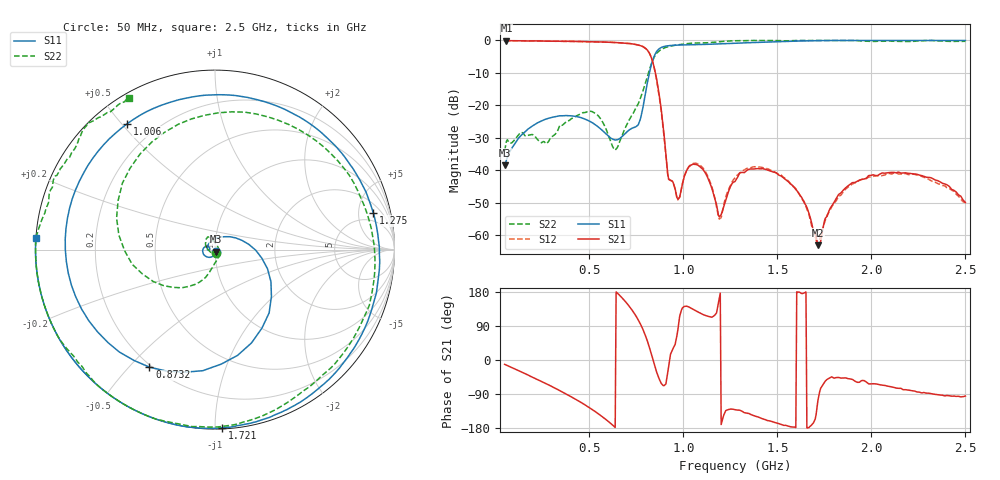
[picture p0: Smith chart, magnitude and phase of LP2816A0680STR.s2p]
!	AVX THIN FILM OPERATION
!	LP2816S High Performance Low Pass Filters
!	P/N LP2816S0680ANTR
! Created  22 November 2016
!Instrument: 	"HEWLETT PACKARD,8720ES,US39172150,7.62 "
# MHz S dB R 50
!  Frq	S11(dB)	S11(deg)	S21(dB)	S21(deg)	S12(dB)	S12(deg)	S22(dB)	S22(deg)
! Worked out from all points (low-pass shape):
!   501 points, 50 MHz to 2.5 GHz, reference 50 ohm
!   highest |S21| = -0.06 dB at 59.8 MHz (marker M1); lowest = -63.1 dB at 1.716 GHz (marker M2)
!   |S21| within 3 dB of the highest: start of sweep to 810.4 MHz
!   lowest |S11| = -38.5 dB at 50 MHz (marker M3), VSWR 1.02, Z = 50.5 - j1.1 ohm
!   |S11| at or under -10 dB: start of sweep to 819.8 MHz
!   |S22| runs from -34.0 to 0.0 dB; largest |S21 - S12| = 0.015
!   S11 on the Smith chart (normalised r, x): 50 MHz: 1.01, -0.02; 873.2 MHz: 0.19, -0.57; 1.006 GHz: 0.10, +0.52; 1.275 GHz: 3.24, +7.36; 1.721 GHz: 0.01, -1.04; 2.5 GHz: -0.00, +0.03
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50  -38.47 -65.8  -0.06 -11.4  -0.07 -11.4  -33.97 -65.4
59.8  -36.78 -73.9  -0.06 -13.5  -0.07 -13.7  -31.05 -76.1
221.5  -25.46 -125.7  -0.14 -50.7  -0.16 -50.6  -30.28 -90.4
461.6  -23.87 172.2  -0.34 -113.5  -0.35 -113.6  -22.38 130.3
642.9  -30.62 174.9  -0.65 179.7  -0.65 179.5  -33.45 8.4
760.5  -25.97 116.5  -1.40 105.9  -1.40 105.4  -19.52 -99.6
819.3  -10.13 -20.1  -3.85 34.1  -3.89 32.9  -9.13 -144.9
868.3  -2.75 -111.8  -15.38 -45.7  -15.77 -46.7  -3.39 128.1
873.2  -2.50 -119.2  -17.25 -51.6  -17.69 -52.4  -3.16 120.5
927.1  -1.58 -179.7  -42.87 -1.2  -42.91 1.8  -1.84 59.4
971.2  -1.42 146.5  -48.88 79.6  -49.08 81.5  -1.33 25.7
1005.5  -1.36 124.9  -41.87 141.4  -41.72 144.8  -1.09 4.6
1103.5  -1.24 75.8  -39.64 120.1  -39.19 121.9  -0.73 -39.8
1196.6  -1.05 39.1  -54.00 176.5  -54.77 178.2  -0.36 -72.3
1275  -0.86 13.0  -43.43 -131.2  -42.27 -132.4  -0.09 -92.0
1520  -0.33 -49.9  -41.73 -170.1  -41.44 -172.3  -0.06 -136.2
1686.6  -0.10 -81.9  -57.29 -169.0  -58.00 -174.1  0.00 -160.0
1716  -0.07 -86.9  -63.12 -106.2  -63.34 -116.6  0.00 -163.8
1720.9  -0.06 -87.7  -62.92 -94.3  -62.27 -106.4  0.00 -164.4
1833.6  0.00 -105.5  -47.10 -47.1  -47.79 -52.0  0.00 -177.3
2093.3  0.00 -140.3  -40.70 -69.5  -40.94 -70.8  -0.16 155.7
2500  0.00 176.3  -49.91 -95.1  -49.81 -96.4  -0.26 119.7
